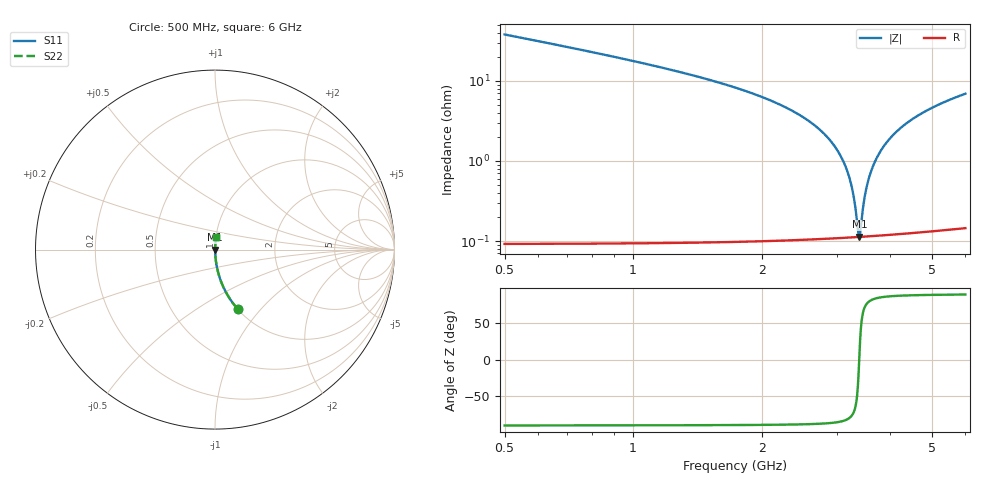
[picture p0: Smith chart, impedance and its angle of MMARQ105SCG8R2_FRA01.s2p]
! MMARQ105SCG8R2_FRA01  S-PARAMETER MODEL  ( General Type )
! Model Generated by TAIYO YUDEN Corporation (http://www.ty-top.com)
! Version 1.0
! TAIYO YUDEN Control No. 200326
! Copyright(c) 2020 TAIYO YUDEN CO.,LTD. All Rights Reserved.
! Product Description (link to TY-COMPAS)
! https://ds.yuden.co.jp/TYCOMPAS/or/detail?pn=MMARQ105SCG8R2CFRA01&u=M
! Products Name : Multilayer Ceramic Capacitors
! Characteristics :
!  Capacitance : 8.2 pF , Rated Voltage : 250V , TCC : CG / C0G
!  Case Size : 1.0 x 0.5 / 0.039 x 0.02 [mm/inch] , Thickness : 0.5 / 0.02 [mm/inch]
!  (Conditions: Temperature = 25 degC , DC Bias Current/Voltage = 0A / 0V)
! External Node Assignments :
!  1  o---| |---o  2
! GND o---------o GND
! Frequency Range : 500MHz  -  6GHz  [ 401 STEP ]
# MHz S RI R 50
! Freq[MHz].  S11 Real  S11 Imag  S21 Real  S21 Imag  S12 Real  S12 Imag  S22 Real  S22 Imag
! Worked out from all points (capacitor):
!   401 points, 500 MHz to 6 GHz, reference 50 ohm
!   read as one part in series: C = 8.2 pF near 527.5 MHz
!   lowest |Z| = 113 mohm at 3.388 GHz (marker M1)
!   series resonance near 3.384 GHz, so ESL is about 270 pH
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500  0.1266 -0.3314  0.8734 0.3314  0.8734 0.3314  0.1266 -0.3314
885  0.0409 -0.1958  0.9591 0.1958  0.9591 0.1958  0.0409 -0.1958
1421.25  0.0134 -0.1109  0.9866 0.1109  0.9866 0.1109  0.0134 -0.1109
2342.5  0.00287 -0.043  0.9971 0.043  0.9971 0.043  0.00287 -0.043
2686.25  0.00176 -0.0266  0.9982 0.0266  0.9982 0.0266  0.00176 -0.0266
2947.5  0.00133 -0.0159  0.9987 0.0159  0.9987 0.0159  0.00133 -0.0159
3126.25  0.00118 -0.00908  0.9988 0.00908  0.9988 0.00908  0.00118 -0.00908
3195  0.00115 -0.00659  0.9989 0.00659  0.9989 0.00659  0.00115 -0.00659
3250  0.00113 -0.00463  0.9989 0.00463  0.9989 0.00463  0.00113 -0.00463
3305  0.00112 -0.00271  0.9989 0.00271  0.9989 0.00271  0.00112 -0.00271
3360  0.00112 -0.000824  0.9989 0.000824  0.9989 0.000824  0.00112 -0.000824
3387.5  0.00112 0.000108  0.9989 -0.000108  0.9989 -0.000108  0.00112 0.000108
3415  0.00113 0.00103  0.9989 -0.00103  0.9989 -0.00103  0.00113 0.00103
3470  0.00114 0.00286  0.9989 -0.00286  0.9989 -0.00286  0.00114 0.00286
3511.25  0.00115 0.00421  0.9988 -0.00421  0.9988 -0.00421  0.00115 0.00421
3566.25  0.00118 0.00599  0.9988 -0.00599  0.9988 -0.00599  0.00118 0.00599
3635  0.00122 0.00818  0.9988 -0.00818  0.9988 -0.00818  0.00122 0.00818
3855  0.0014 0.0149  0.9986 -0.0149  0.9986 -0.0149  0.0014 0.0149
4171.25  0.00179 0.024  0.9982 -0.024  0.9982 -0.024  0.00179 0.024
4570  0.00248 0.0348  0.9975 -0.0348  0.9975 -0.0348  0.00248 0.0348
5092.5  0.00363 0.0478  0.9964 -0.0478  0.9964 -0.0478  0.00363 0.0478
6000  0.00618 0.0686  0.9938 -0.0686  0.9938 -0.0686  0.00618 0.0686
